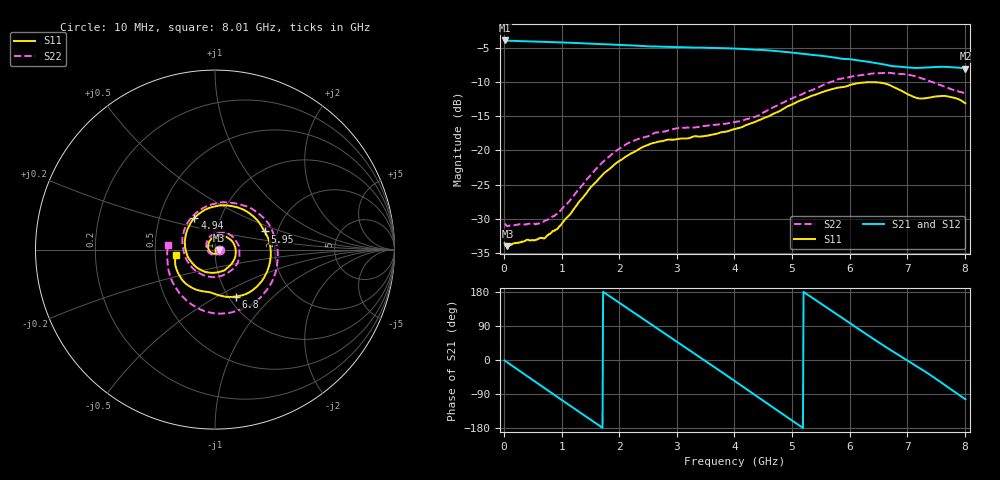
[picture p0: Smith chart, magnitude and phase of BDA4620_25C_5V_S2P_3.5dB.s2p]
!Agilent Technologies,E5071B,MY42404982,A.09.10
!Date: Wed May 06 08:58:49 2026
!Data & Calibration Information:
!Freq	S11:SOLT2(ON)	S21:SOLT2(ON)	S12:SOLT2(ON)	S22:SOLT2(ON)
# Hz S RI R 50
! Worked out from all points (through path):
!   801 points, 10 MHz to 8.01 GHz, reference 50 ohm
!   highest |S21| = -3.95 dB at 10 MHz (marker M1); lowest = -8.1 dB at 8.01 GHz (marker M2)
!   group delay of S21, straight-line fit = 286 ps
!   lowest |S11| = -34.0 dB at 60 MHz (marker M3), VSWR 1.04, Z = 52 - j0.242 ohm
!   |S11| at or under -10 dB: start of sweep to end of sweep
!   |S22| runs from -31.0 to -8.7 dB; largest |S21 - S12| = 0.0028
!   S11 on the Smith chart (normalised r, x): 10 MHz: 1.04, -0.00; 4.94 GHz: 0.75, +0.28; 5.95 GHz: 1.71, +0.38; 6.8 GHz: 1.08, -0.61; 8.01 GHz: 0.64, -0.04
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1e7  0.0209 -0.00143  0.6348 -0.0136  0.636 -0.0138  0.0293 -0.00198
6e7  0.0199 -0.00232  0.6283 -0.0728  0.6296 -0.0737  0.0278 -0.00375
3.7e8  0.0165 -0.0144  0.4849 -0.396  0.4855 -0.3971  0.0204 -0.0204
7.3e8  -0.00331 -0.0232  0.1391 -0.6037  0.1388 -0.6047  -0.00647 -0.0302
1.03e9  -0.0276 -0.0122  -0.1932 -0.5817  -0.1937 -0.5827  -0.0356 -0.0147
1.35e9  -0.0389 0.0213  -0.4758 -0.3754  -0.4761 -0.3761  -0.0486 0.0265
1.64e9  -0.0225 0.0574  -0.5926 -0.0859  -0.5933 -0.086  -0.03 0.0702
1.93e9  0.0179 0.0777  -0.549 0.2185  -0.5498 0.2192  0.0183 0.0963
2.32e9  0.0821 0.0584  -0.273 0.5129  -0.2737 0.5137  0.0959 0.0737
2.68e9  0.116 -0.00404  0.086 0.5666  0.0868 0.567  0.1353 0.00579
3.07e9  0.0907 -0.082  0.4255 0.3761  0.4271 0.3757  0.1188 -0.0854
3.38e9  0.0365 -0.1206  0.5555 0.0937  0.5564 0.0926  0.057 -0.1371
3.69e9  -0.0331 -0.1281  0.5163 -0.2147  0.5161 -0.2158  -0.0306 -0.151
4.01e9  -0.1069 -0.0955  0.3095 -0.4591  0.3093 -0.4599  -0.1206 -0.1073
4.46e9  -0.1672 0.0199  -0.1223 -0.5278  -0.1227 -0.5281  -0.1809 0.0338
4.94e9  -0.1142 0.1775  -0.4655 -0.2327  -0.4669 -0.2327  -0.0937 0.2139
5.35e9  0.045 0.2471  -0.4794 0.1356  -0.4797 0.1364  0.0922 0.2602
5.95e9  0.2761 0.1014  -0.1056 0.4528  -0.1051 0.4536  0.3316 0.0708
6.68e9  0.173 -0.2473  0.3643 0.203  0.3657 0.2029  0.2083 -0.3041
6.8e9  0.1145 -0.2614  0.3905 0.1271  0.392 0.1267  0.1437 -0.3333
7.36e9  -0.0698 -0.2312  0.328 -0.235  0.3286 -0.2361  -0.1613 -0.2811
8.01e9  -0.2188 -0.0319  -0.0934 -0.3846  -0.0938 -0.3859  -0.2598 0.0265
